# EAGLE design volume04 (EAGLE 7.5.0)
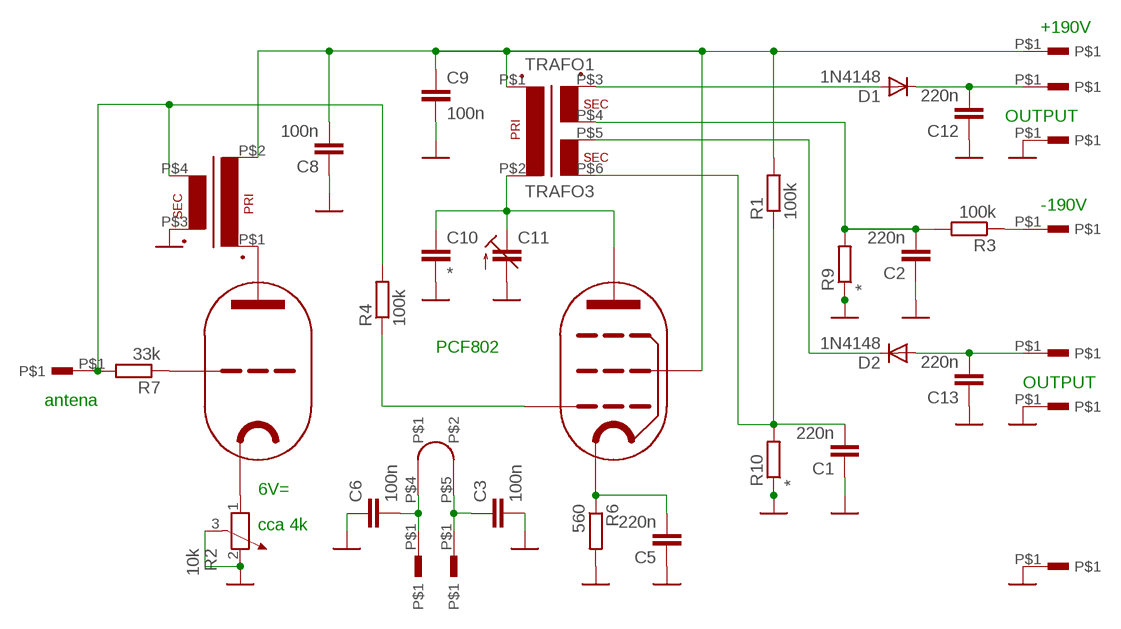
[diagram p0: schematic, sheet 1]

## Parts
C1  220n  C-EU050-024X044  [C050-024X044]
C2  220n  C-EU050-024X044  [C050-024X044]
C3  100n  C-EU050-024X044  [C050-024X044]
C5  220n  C-EU050-024X044  [C050-024X044]
C6  100n  C-EU050-024X044  [C050-024X044]
C8  100n  C-EU075-032X103  [C075-032X103]
C9  100n  C-EU075-032X103  [C075-032X103]
C10  *  C-EU075-032X103  [C075-032X103]
C11  C-TRIMMCT10MM  [CTRIM10MM]
C12  220n  C-EU050-024X044  [C050-024X044]
C13  220n  C-EU050-024X044  [C050-024X044]
D1  1N4148  1N4004  [DO41-10]
D2  1N4148  1N4004  [DO41-10]
R1  100k  R-EU_0207/10  [0207/10]
R2  10k  POTENTIOMETER_PT-10  [PT-10]
R3  100k  R-EU_0207/10  [0207/10]
R4  100k  R-EU_0207/10  [0207/10]
R6  560  R-EU_0207/10  [0207/10]
R7  33k  R-EU_0207/10  [0207/10]
R9  *  R-EU_0207/10  [0207/10]
R10  *  R-EU_0207/10  [0207/10]
TRAFO1  TRAFO3  [TRAFO_3]
U$1  PCF802  PCF82  [NOVAL02]
U$2  PIN  [PIN]
U$4  PIN  [PIN]
U$5  PIN  [PIN]
U$6  PIN  [PIN]
U$7  PIN  [PIN]
U$8  PIN  [PIN]
U$9  TRAFO_18  [EI18]
U$10  PIN  [PIN]
U$12  PIN  [PIN]
U$13  PIN  [PIN]
U$14  PIN  [PIN]

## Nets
GND: C1.1 C2.1 C3.2 C5.1 C6.1 C8.1 C9.2 C10.2 C11.1A(A) C11.1B(A) C12.1 C13.1 R2.2 R2.3 R6.2 R9.1 R10.1 U$6.P$1 U$9.P$3(S1) U$13.P$1 U$14.P$1
N$1: U$1.P$1(A) U$9.P$1(P1)
N$2: C10.1 C11.2(E) TRAFO1.P$2(P2) U$1.P$6(A)
N$3: R4.1 U$1.P$2(G1)
N$4: C5.2 R6.1 U$1.P$7(K)
N$5: C8.2 C9.1 R1.2 TRAFO1.P$1(P1) U$1.P$3(G2) U$4.P$1 U$9.P$2(P2)
N$6: D1.A TRAFO1.P$3(S1)
N$7: R7.1 U$1.P$9(G1)
N$8: D2.C TRAFO1.P$5(S3)
N$9: R4.2 R7.2 U$2.P$1 U$9.P$4(S2)
N$10: C6.2 U$1.P$4 U$7.P$1
N$11: C3.1 U$1.P$5 U$8.P$1
N$12: C1.2 R1.1 R10.2 TRAFO1.P$6(S4)
N$13: R2.1 U$1.P$8(K)
N$14: C2.2 R3.2 R9.2 TRAFO1.P$4(S2)
N$15: C12.2 D1.C U$10.P$1
N$16: C13.2 D2.A U$12.P$1
N$19: R3.1 U$5.P$1

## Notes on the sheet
- +190V
- OUTPUT
- -190V
- PCF802
- OUTPUT
- antena
- 6V=
- cca 4k

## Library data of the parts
C1-C3 C5 C6 C8-C10 C12 C13 = rcl:C-EU: CAPACITOR, European symbol
C11 = rcl:C-TRIMM: Trimm capacitor
D1 D2 = diode:1N4004: DIODE
R1 R3 R4 R6 R7 R9 R10 = rcl:R-EU_: RESISTOR, European symbol
R2 = rcl:POTENTIOMETER_: Potentiometer
TRAFO1 = trafo_ferit:TRAFO3
U$1 = lampy03:PCF82
U$2 U$4-U$8 U$10 U$12-U$14 = lampy04:PIN
U$9 = trafo_ferit:TRAFO_18

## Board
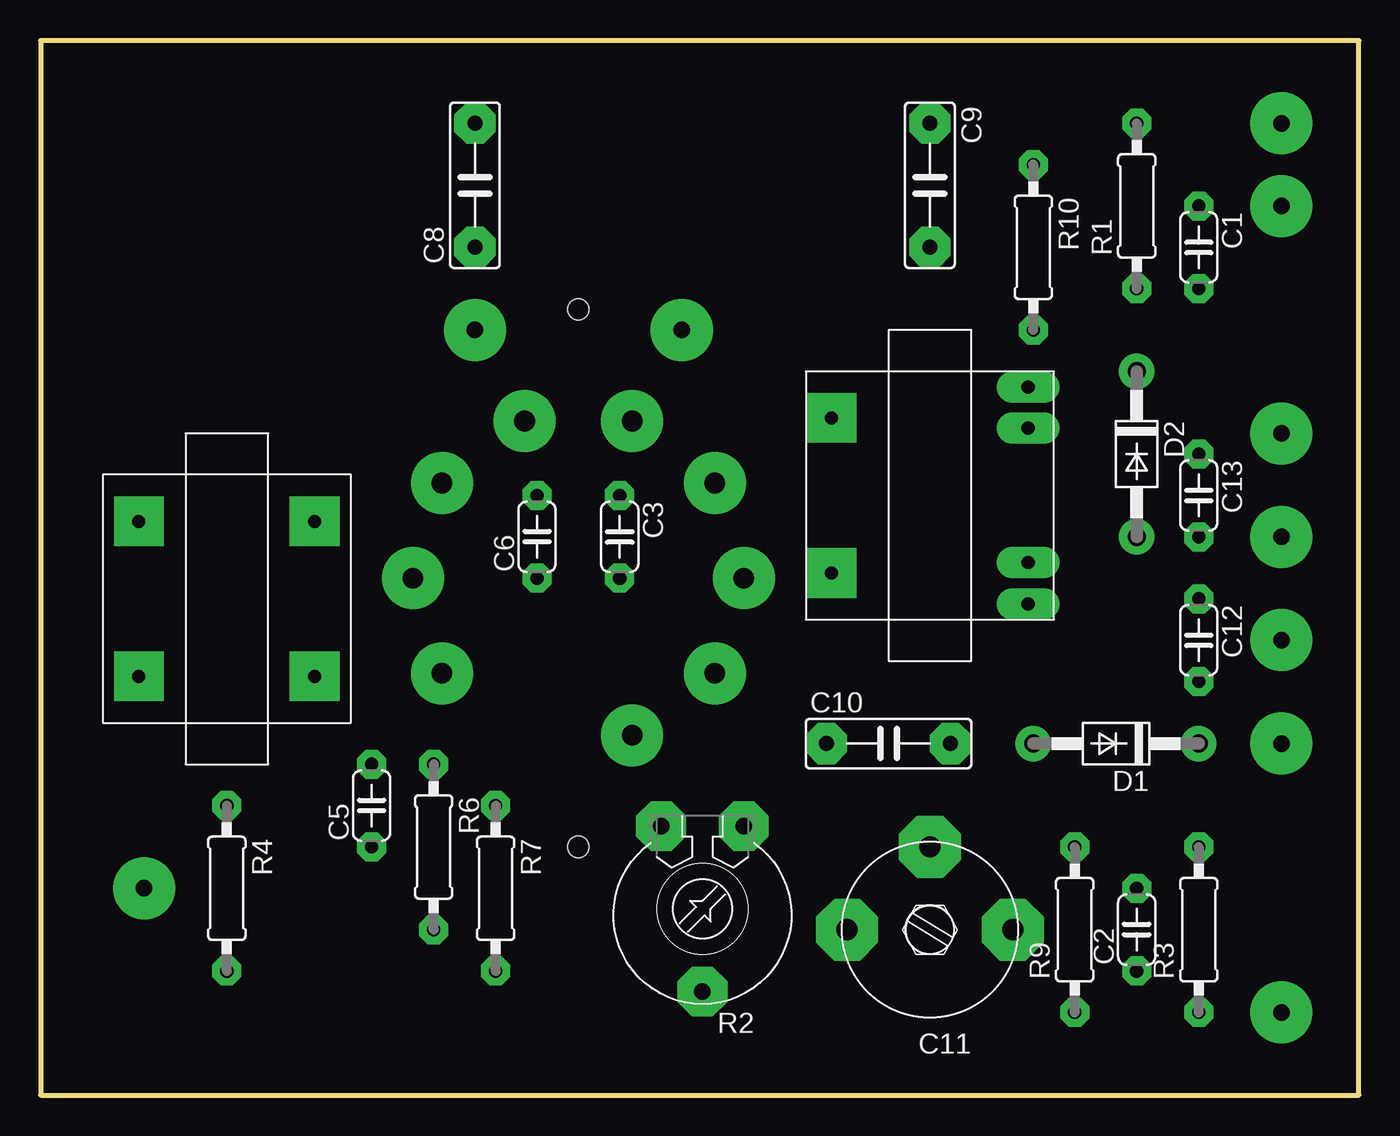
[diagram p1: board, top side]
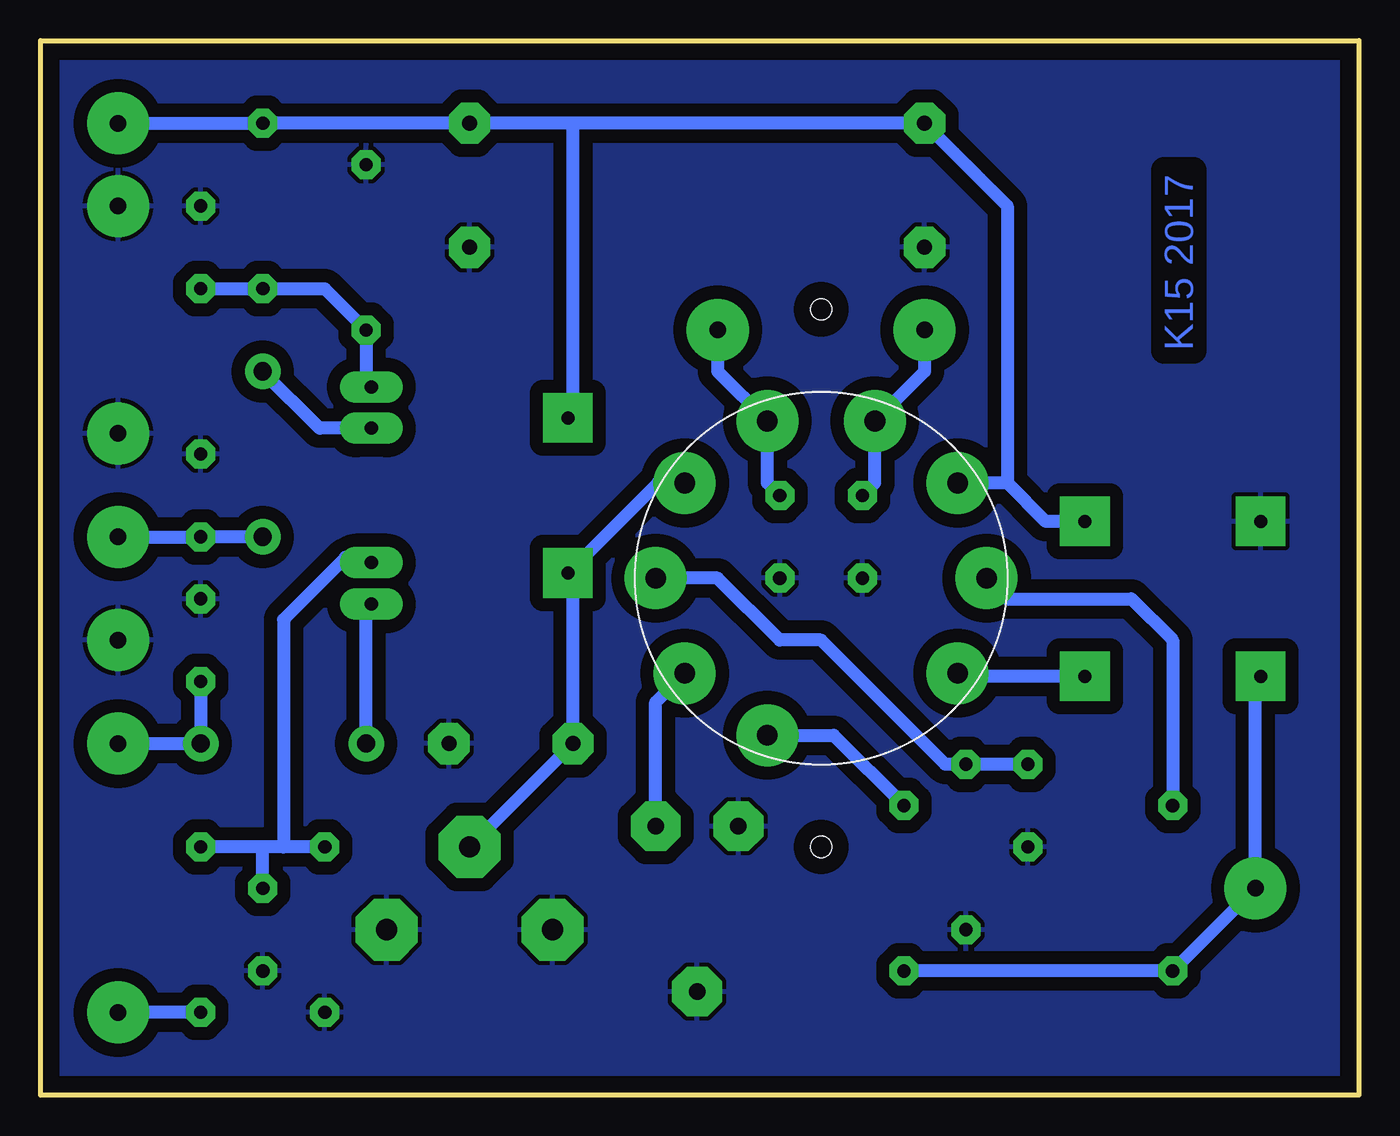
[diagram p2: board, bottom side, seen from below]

Size 80.95 x 64.76 mm. Coordinates in mm from the lower left corner, seen from the top.
Outline: 0,0 80.95,0 80.95,64.76 0,64.76 0,0
Copper layers (1*16): Top 0.035mm / dielectric 1.5mm / Bottom 0.035mm
Design rules "default": minimum track width 10mil, minimum drill 24mil, track to track 8mil, track to pad 8mil, pad to pad 8mil, via to via 8mil, smd to smd 8mil, copper to edge 40mil, drill to drill 8mil, minimum pad ring 10mil, minimum via ring 8mil, stop-mask expansion 4mil, vias tented up to drill 0mil, thermal gap 10mil
Holes 1.3 mm at 33.02,48.26 33.02,15.24

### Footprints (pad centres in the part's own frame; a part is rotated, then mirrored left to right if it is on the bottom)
C050-024X044 = drill 0.813 pad 1.778 octagon: 1 -2.54,0; 2 2.54,0
C075-032X103 = drill 0.914 pad 2.54 octagon: 1 -3.81,0; 2 3.81,0
CTRIM10MM = drill 1.3 pad 3.81 octagon: 1A -5.088,0; 1B 5.088,0; 2 0,-5.088
DO41-10 = drill 1.118 pad 2.184: A 5.08,0; C -5.08,0
0207/10 = drill 0.813 pad 1.778 octagon: 1 -5.08,0; 2 5.08,0
PT-10 = drill 1.016 pad 3.048 octagon: 1 -2.54,-5.08; 2 2.54,-5.08; 3 0,5.08
TRAFO_3 = drill 0.8 pad 3.048 square: P$1 -4.763,-6.032; P$2 4.763,-6.032 | drill 0.8 pad 1.93 long: P$3 6.668,6.032; P$4 4.128,6.032; P$5 -4.128,6.032; P$6 -6.668,6.032
NOVAL02 = drill 1.27 pad 3.81: P$1 8.382,-5.842; P$2 10.16,0; P$3 8.382,5.842; P$4 3.302,9.652; P$5 -3.302,9.652; P$6 -8.382,5.842; P$7 -10.16,0; P$8 -8.382,-5.842; P$9 -3.302,-9.652
PIN = drill 1.016 pad 3.81: P$1 0,0
EI18 = drill 0.8 pad 3.048 square: P$1 -4.763,-5.397; P$2 4.763,-5.397; P$3 4.763,5.397; P$4 -4.763,5.397

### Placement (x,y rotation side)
C1  71.12,52.07 270 top
C2  67.31,10.16 90 top
C3  35.56,34.29 270 top
C5  20.32,17.78 90 top
C6  30.48,34.29 90 top
C8  26.67,55.88 90 top
C9  54.61,55.88 270 top
C10  52.07,21.59 0 top
C11  54.61,10.16 180 top
C12  71.12,27.94 270 top
C13  71.12,36.83 270 top
D1  66.04,21.59 180 top
D2  67.31,39.37 270 top
R1  67.31,54.61 90 top
R2  40.64,11.43 180 top
R3  71.12,10.16 90 top
R4  11.43,12.7 270 top
R6  24.13,15.24 270 top
R7  27.94,12.7 270 top
R9  63.5,10.16 90 top
R10  60.96,52.07 270 top
TRAFO1  54.61,36.83 270 top
U$1  33.02,31.75 0 bottom
U$2  6.35,12.7 0 top
U$4  76.2,59.69 0 top
U$5  76.2,5.08 0 top
U$6  76.2,54.61 0 top
U$7  26.67,46.99 0 top
U$8  39.37,46.99 0 top
U$9  11.43,30.48 90 top
U$10  76.2,21.59 0 top
U$12  76.2,34.29 0 top
U$13  76.2,40.64 0 top
U$14  76.2,27.94 0 top

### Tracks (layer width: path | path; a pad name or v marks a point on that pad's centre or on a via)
GND
  pour Bottom (isolate 0.813): 0,64.77 81.28,64.77 81.28,0 0,0
N$1
  Bottom 0.813: U$9.P$1 24.45,25.72 U$1.P$1
N$2
  Bottom 0.813: U$1.P$6 43.05,37.59 TRAFO1.P$2 48.26,31.11 C10.1 C11.2
N$3
  Bottom 0.813: U$1.P$2 21.59,30.48 13.97,30.48 11.43,27.94 R4.1
N$4
  Bottom 0.813: C5.2 R6.1 25.4,20.32 33.02,27.94 35.56,27.94 39.37,31.75 U$1.P$7
N$5
  Bottom 0.813: 21.59,37.59 21.59,54.61 C8.2 48.26,59.69 | 21.59,37.59 U$1.P$3 | U$9.P$2 19.24,35.24 21.59,37.59 | 48.26,59.69 C9.1 R1.2 U$4.P$1 | TRAFO1.P$1 48.26,41.59 48.26,59.69
N$6
  Bottom 0.813: D1.A 60.96,29.85 TRAFO1.P$3
N$7
  Bottom 0.813: U$1.P$9 32.26,22.1 R7.1
N$8
  Bottom 0.813: TRAFO1.P$5 63.82,40.96 D2.C
N$9
  Bottom 0.813: R7.2 R4.2 U$2.P$1 6.35,25.4 U$9.P$4
N$10
  Bottom 0.813: C6.2 29.72,37.59 U$1.P$4 26.67,44.45 U$7.P$1
N$11
  Bottom 0.813: C3.1 36.32,37.59 U$1.P$5 39.37,44.45 U$8.P$1
N$12
  Bottom 0.813: C1.2 R1.1 63.5,49.53 R10.2 60.96,43.18 TRAFO1.P$6
N$13
  Bottom 0.813: R2.1 43.18,24.13 U$1.P$8
N$14
  Bottom 0.813: R9.2 66.04,15.24 | 66.04,15.24 67.31,15.24 | 67.31,15.24 R3.2 | TRAFO1.P$4 60.96,33.02 62.23,33.02 66.04,29.21 66.04,15.24 | C2.2 67.31,15.24
N$15
  Bottom 0.813: C12.2 D1.C U$10.P$1
N$16
  Bottom 0.813: D2.A C13.2 U$12.P$1
N$19
  Bottom 0.813: R3.1 U$5.P$1

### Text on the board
Bottom: K15 2017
